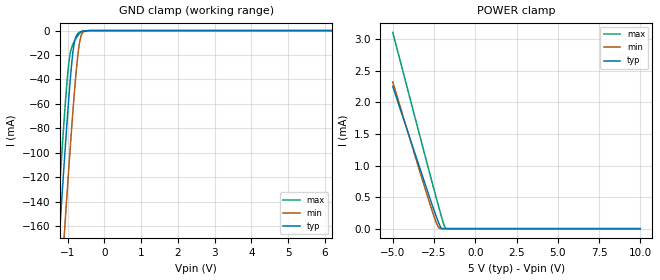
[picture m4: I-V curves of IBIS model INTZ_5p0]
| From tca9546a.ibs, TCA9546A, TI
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|   Model
[Model]   INTZ_5p0
Model_type   Input
Vinl = 1.5
Vinh = 3.5
|   typ   min   max
C_comp   1.378pF   1.292pF   1.466pF
[Voltage Range]   5   4.5   5.5
[Temperature Range]   27   125   -40
[Power Clamp Reference]   5   4.5   5.5
[GND Clamp Reference]   -0   -0   -0
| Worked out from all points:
|   GND clamp passes 1 mA (typ) near -0.65 V on its own axis
|   POWER clamp passes 1 mA (typ) near -3.41 V on its own axis
[GND Clamp]
|   Voltage   I(typ)   I(min)   I(max)
-5V       -2.025A    -2.08A     -1.991A
-1.43V    -266.3mA   -326.9mA   -228.4mA
-1.25V    -181.4mA   -242.1mA   -143.6mA
-1.145V   -133.2mA   -193.4mA   -95.99mA
-1.1V     -112.9mA   -172.9mA   -76.42mA
-1.055V   -93.1mA    -152.6mA   -57.8mA
-965mV    -55.49mA   -112.8mA   -26.77mA
-845mV    -15.74mA   -62.98mA   -10.69mA
-725mV    -2.715mA   -21.75mA   -4.331mA
-620mV    -647.4uA   -3.376mA   -1.122mA
-380mV    -4.624uA   -12.11uA   -4.663uA
9.985V    0A         0A         0A
[POWER Clamp]
|   Voltage   I(typ)   I(min)   I(max)
-5V       2.254mA    2.322mA    3.108mA
-3.155V   796.5uA    731.5uA    1.266mA
-2.435V   243.9uA    146uA      556.9uA
-2.255V   115.1uA    32.65uA    383uA
-2.18V    66.39uA    8.214uA    311.6uA
-2.09V    19.56uA    740.7nA    227.3uA
-1.91V    13.04nA    0A         69.76uA
-1.805V   0A         0A         7.917uA
9.985V    0A         0A         0A
